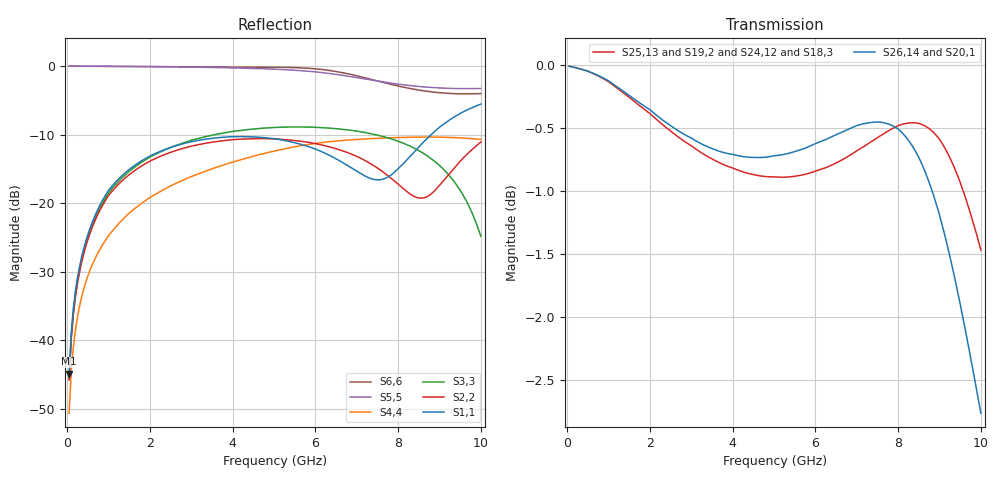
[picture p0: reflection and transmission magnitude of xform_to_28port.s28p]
! Created Tue Jan 21 22:45:03 2014
! 28 Port Network Data from SP1.SP block
! freq  magS1_1  angS1_1  magS1_2  angS1_2  magS1_3  angS1_3  magS1_4  angS1_4
!  magS1_5  angS1_5  magS1_6  angS1_6  magS1_7  angS1_7  magS1_8  angS1_8
!  magS1_9  angS1_9  magS1_10  angS1_10  magS1_11  angS1_11  magS1_12  angS1_12
!  magS1_13  angS1_13  magS1_14  angS1_14  magS1_15  angS1_15  magS1_16  angS1_16
!  magS1_17  angS1_17  magS1_18  angS1_18  magS1_19  angS1_19  magS1_20  angS1_20
!  magS1_21  angS1_21  magS1_22  angS1_22  magS1_23  angS1_23  magS1_24  angS1_24
!  magS1_25  angS1_25  magS1_26  angS1_26  magS1_27  angS1_27  magS1_28  angS1_28
!  magS2_1  angS2_1  magS2_2  angS2_2  magS2_3  angS2_3  magS2_4  angS2_4
!  magS2_5  angS2_5  magS2_6  angS2_6  magS2_7  angS2_7  magS2_8  angS2_8
!  magS2_9  angS2_9  magS2_10  angS2_10  magS2_11  angS2_11  magS2_12  angS2_12
!  magS2_13  angS2_13  magS2_14  angS2_14  magS2_15  angS2_15  magS2_16  angS2_16
!  magS2_17  angS2_17  magS2_18  angS2_18  magS2_19  angS2_19  magS2_20  angS2_20
!  magS2_21  angS2_21  magS2_22  angS2_22  magS2_23  angS2_23  magS2_24  angS2_24
!  magS2_25  angS2_25  magS2_26  angS2_26  magS2_27  angS2_27  magS2_28  angS2_28
!  magS3_1  angS3_1  magS3_2  angS3_2  magS3_3  angS3_3  magS3_4  angS3_4
!  magS3_5  angS3_5  magS3_6  angS3_6  magS3_7  angS3_7  magS3_8  angS3_8
!  magS3_9  angS3_9  magS3_10  angS3_10  magS3_11  angS3_11  magS3_12  angS3_12
!  magS3_13  angS3_13  magS3_14  angS3_14  magS3_15  angS3_15  magS3_16  angS3_16
!  magS3_17  angS3_17  magS3_18  angS3_18  magS3_19  angS3_19  magS3_20  angS3_20
!  magS3_21  angS3_21  magS3_22  angS3_22  magS3_23  angS3_23  magS3_24  angS3_24
!  magS3_25  angS3_25  magS3_26  angS3_26  magS3_27  angS3_27  magS3_28  angS3_28
!  magS4_1  angS4_1  magS4_2  angS4_2  magS4_3  angS4_3  magS4_4  angS4_4
!  magS4_5  angS4_5  magS4_6  angS4_6  magS4_7  angS4_7  magS4_8  angS4_8
!  magS4_9  angS4_9  magS4_10  angS4_10  magS4_11  angS4_11  magS4_12  angS4_12
!  magS4_13  angS4_13  magS4_14  angS4_14  magS4_15  angS4_15  magS4_16  angS4_16
!  magS4_17  angS4_17  magS4_18  angS4_18  magS4_19  angS4_19  magS4_20  angS4_20
!  magS4_21  angS4_21  magS4_22  angS4_22  magS4_23  angS4_23  magS4_24  angS4_24
!  magS4_25  angS4_25  magS4_26  angS4_26  magS4_27  angS4_27  magS4_28  angS4_28
!  magS5_1  angS5_1  magS5_2  angS5_2  magS5_3  angS5_3  magS5_4  angS5_4
!  magS5_5  angS5_5  magS5_6  angS5_6  magS5_7  angS5_7  magS5_8  angS5_8
!  magS5_9  angS5_9  magS5_10  angS5_10  magS5_11  angS5_11  magS5_12  angS5_12
!  magS5_13  angS5_13  magS5_14  angS5_14  magS5_15  angS5_15  magS5_16  angS5_16
!  magS5_17  angS5_17  magS5_18  angS5_18  magS5_19  angS5_19  magS5_20  angS5_20
!  magS5_21  angS5_21  magS5_22  angS5_22  magS5_23  angS5_23  magS5_24  angS5_24
!  magS5_25  angS5_25  magS5_26  angS5_26  magS5_27  angS5_27  magS5_28  angS5_28
!  magS6_1  angS6_1  magS6_2  angS6_2  magS6_3  angS6_3  magS6_4  angS6_4
!  magS6_5  angS6_5  magS6_6  angS6_6  magS6_7  angS6_7  magS6_8  angS6_8
!  magS6_9  angS6_9  magS6_10  angS6_10  magS6_11  angS6_11  magS6_12  angS6_12
!  magS6_13  angS6_13  magS6_14  angS6_14  magS6_15  angS6_15  magS6_16  angS6_16
!  magS6_17  angS6_17  magS6_18  angS6_18  magS6_19  angS6_19  magS6_20  angS6_20
!  magS6_21  angS6_21  magS6_22  angS6_22  magS6_23  angS6_23  magS6_24  angS6_24
!  magS6_25  angS6_25  magS6_26  angS6_26  magS6_27  angS6_27  magS6_28  angS6_28
!  magS7_1  angS7_1  magS7_2  angS7_2  magS7_3  angS7_3  magS7_4  angS7_4
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# ghz S ma R 50
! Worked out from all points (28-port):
!   200 points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, 50 MHz to 10 GHz, reference 50 ohm
!   strongest paths, dB at 50 MHz, 2.55 GHz, 5.05 GHz, 7.55 GHz, 10 GHz:
!     S26,14: 0.0, -0.5, -0.7, -0.5, -2.8
!     S20,1: 0.0, -0.5, -0.7, -0.5, -2.8
!     S25,13: 0.0, -0.5, -0.9, -0.6, -1.5
!     S19,2: 0.0, -0.5, -0.9, -0.6, -1.4
!     S24,12: 0.0, -0.6, -1.1, -0.9, -0.7
!     S18,3: 0.0, -0.6, -1.1, -0.9, -0.7
!   lowest |S11| = -44.8 dB at 50 MHz (marker M1), VSWR 1.01, Z = 50.5 + j0.34 ohm
!   |S11| at or under -10 dB: start of sweep to 8.795 GHz
